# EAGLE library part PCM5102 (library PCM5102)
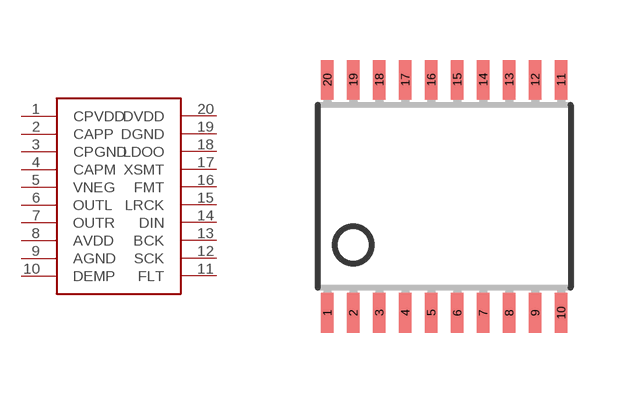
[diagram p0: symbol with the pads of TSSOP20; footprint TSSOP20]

Designator prefix -

## PCM5102  [TSSOP20]
1  CPVDD
2  CAPP
3  CPGND
4  CAPM
5  VNEG
6  OUTL
7  OUTR
8  AVDD
9  AGND
10  DEMP
11  FLT
12  SCK
13  BCK
14  DIN
15  LRCK
16  FMT
17  XSMT
18  LDOO
19  DGND
20  DVDD

## Footprint TSSOP20 (pad centres in mm)
smd 0.305 x 0.991: 1 -2.925,-2.918; 2 -2.275,-2.918; 3 -1.625,-2.918; 4 -0.975,-2.918; 5 -0.325,-2.918; 6 0.325,-2.918; 7 0.975,-2.918; 8 1.625,-2.918; 9 2.275,-2.918; 10 2.925,-2.918; 11 2.925,2.918; 12 2.275,2.918; 13 1.625,2.918; 14 0.975,2.918; 15 0.325,2.918; 16 -0.325,2.918; 17 -0.975,2.918; 18 -1.625,2.918; 19 -2.275,2.918; 20 -2.925,2.918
